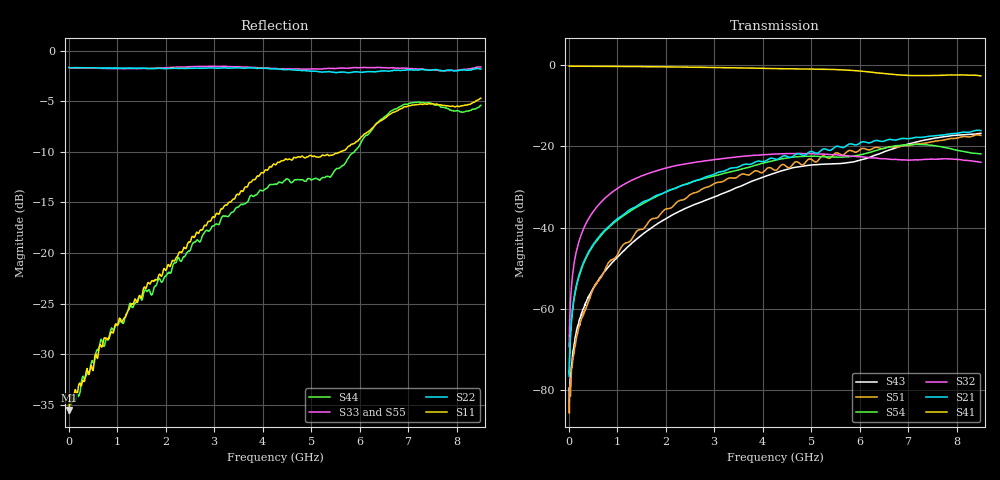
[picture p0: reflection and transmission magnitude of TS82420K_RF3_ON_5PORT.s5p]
!Created with skrf (http://scikit-rf.org).
# GHz S RI R 50.0
!freq ReS11 ImS11 ReS12 ImS12 ReS13 ImS13
! ReS14 ImS14 ReS15 ImS15
! ReS21 ImS21 ReS22 ImS22 ReS23 ImS23
! ReS24 ImS24 ReS25 ImS25
! ReS31 ImS31 ReS32 ImS32 ReS33 ImS33
! ReS34 ImS34 ReS35 ImS35
! ReS41 ImS41 ReS42 ImS42 ReS43 ImS43
! ReS44 ImS44 ReS45 ImS45
! ReS51 ImS51 ReS52 ImS52 ReS53 ImS53
! ReS54 ImS54 ReS55 ImS55
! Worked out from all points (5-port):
!   1601 points, 10 MHz to 8.5 GHz, reference 50 ohm
!   strongest paths, dB at 10 MHz, 2.132 GHz, 4.255 GHz, 6.378 GHz, 8.5 GHz:
!     S41: -0.2, -0.4, -0.8, -1.9, -2.6
!     S21: -76.6, -30.5, -23.1, -18.5, -16.1
!     S32: -69.3, -24.9, -21.9, -22.9, -23.9
!     S54: -76.0, -30.6, -23.4, -20.8, -21.8
!     S51: -83.3, -35.0, -25.9, -20.2, -17.3
!     S43: -83.0, -36.9, -26.5, -21.9, -16.8
!   lowest |S11| = -35.5 dB at 10 MHz (marker M1), VSWR 1.03, Z = 51.7 + j0.0222 ohm
!   |S11| at or under -10 dB: start of sweep to 5.601 GHz
